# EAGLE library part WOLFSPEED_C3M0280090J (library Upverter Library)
Silicon Carbide Power MOSFET N-Channel 11A (Tc) 50W (Tc) Surface Mount D2PAK-7
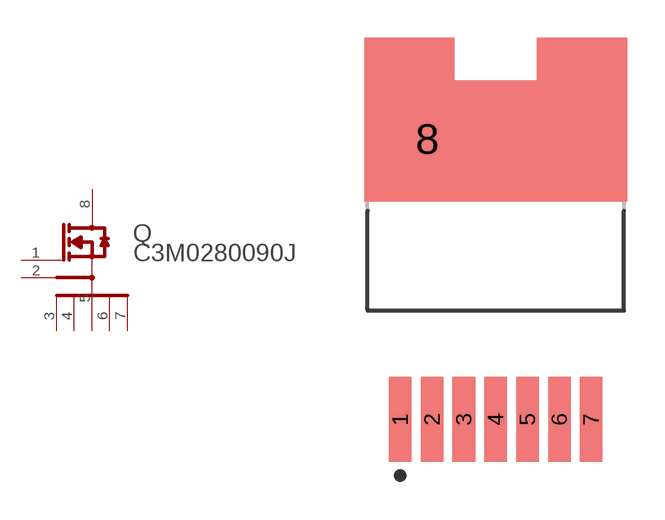
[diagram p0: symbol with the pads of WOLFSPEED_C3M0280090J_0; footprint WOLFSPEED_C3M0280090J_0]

Designator prefix Q

## WOLFSPEED_C3M0280090JWOLFSPEED_C3M0280090J_0_0 (MF: Wolfspeed; MPN: C3M0280090J; automotive: No; centroid_not_specified: Yes; continuous_drain_current: 11A; datasheet: https://assets.wolfspeed.com/uploads/2020/12/C3M0280090J.pdf; depletion_mode: False; device_class_L1: Discrete Semiconductors; device_class_L2: Transistors; device_class_L3: MOSFETs; digikey_description: SICFET N-CH 900V 11A D2PAK-7; digikey_part_number: C3M0280090J-ND; drain_to_source_breakdown_voltage: 900V; drain_to_source_resistance: 320mΩ; drain_to_source_voltage: 900V; footprint_variant_name_0: Recommended_Land_Pattern; gate_charge_at_vgs: 10nC @ 15V; gate_to_source_voltage: 18V; height: 4.82mm; input_capacitace_at_vds: 204pF @ 600V; lead_free: Yes; max_junction_temp: +150°C; mfg_package_ident: TO-263-7; mfg_package_ident_component_id: d2de6d38281de76c; mfg_package_ident_date: 0; mfg_package_ident_rev: 0; mouser_part_number: 941-C3M0280090J; number_of_N_channels: 1; number_of_channels: 1; package: TO-263-7; power_dissipation: 49W; prefix: Q; pulse_drain_current: 22A; reverse_recovery_charge: 39nC; reverse_recovery_time: 8ns; rohs: Yes; rthja_max: 40°C/W; standoff_height: 0mm; technology: SiC; temperature_range_high: +150°C; temperature_range_low: -55°C; threshold_vgs_max: 3.5V; threshold_vgs_min: 1.8V; transconductance: 3.6S; turn_off_delay_time: 7ns; turn_on_delay_time: 4ns; typ_forward_diode_voltage: 4.8V; verification_version: 0.0.0.3)  [WOLFSPEED_C3M0280090J_0]
1  GATE  pas
2  DRIVER_SOURCE  pas
3  1_POWER_SOURCE  pas
4  2_POWER_SOURCE  pas
5  3_POWER_SOURCE  pas
6  4_POWER_SOURCE  pas
7  5_POWER_SOURCE  pas
8  DRAIN  pas

## Footprint WOLFSPEED_C3M0280090J_0 (pad centres in mm)
Silicon Carbide Power MOSFET N-Channel 11A (Tc) 50W (Tc) Surface Mount D2PAK-7
smd 0.9 x 3.4: 1 -3.81,-6.764; 2 -2.54,-6.764; 3 -1.27,-6.764; 4 0,-6.764; 5 1.27,-6.764; 6 2.54,-6.764; 7 3.81,-6.764
smd 4.505 x 4.505: 8 -2.737,4.429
